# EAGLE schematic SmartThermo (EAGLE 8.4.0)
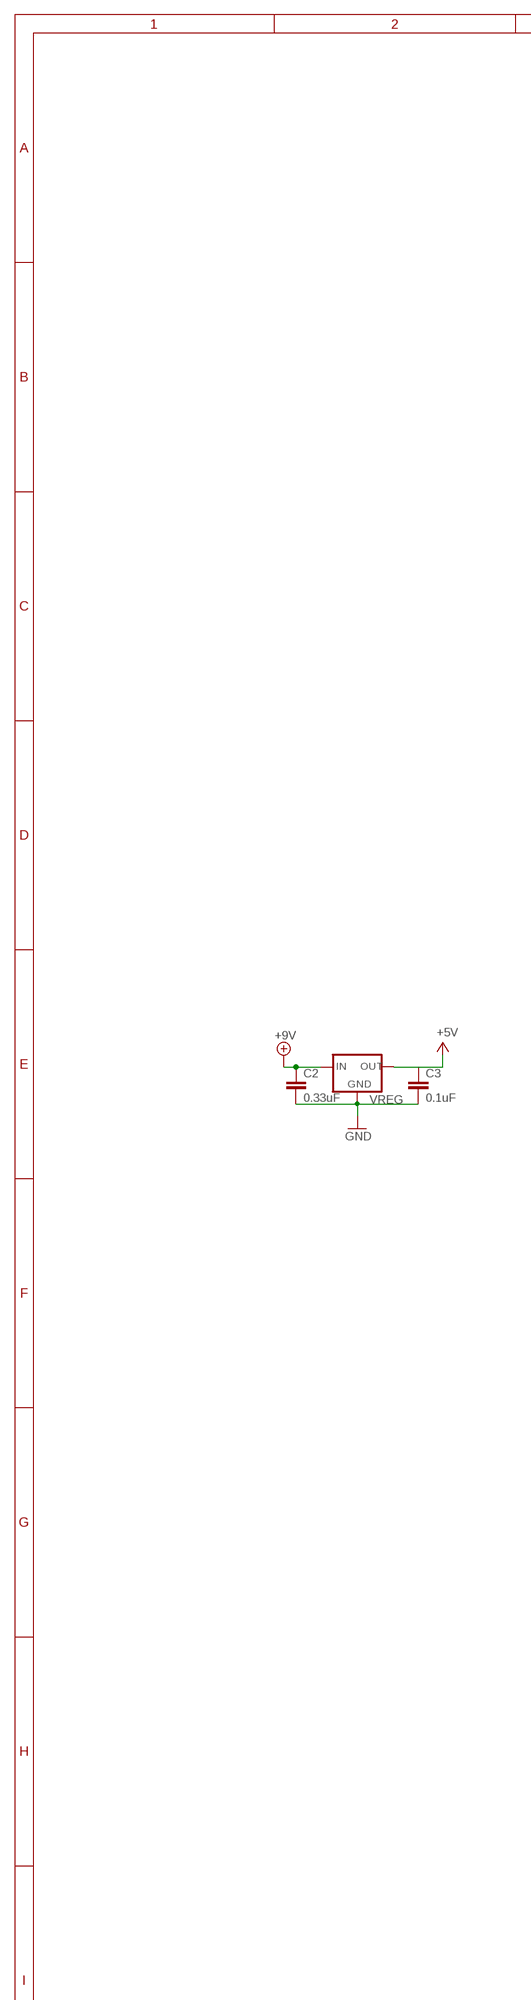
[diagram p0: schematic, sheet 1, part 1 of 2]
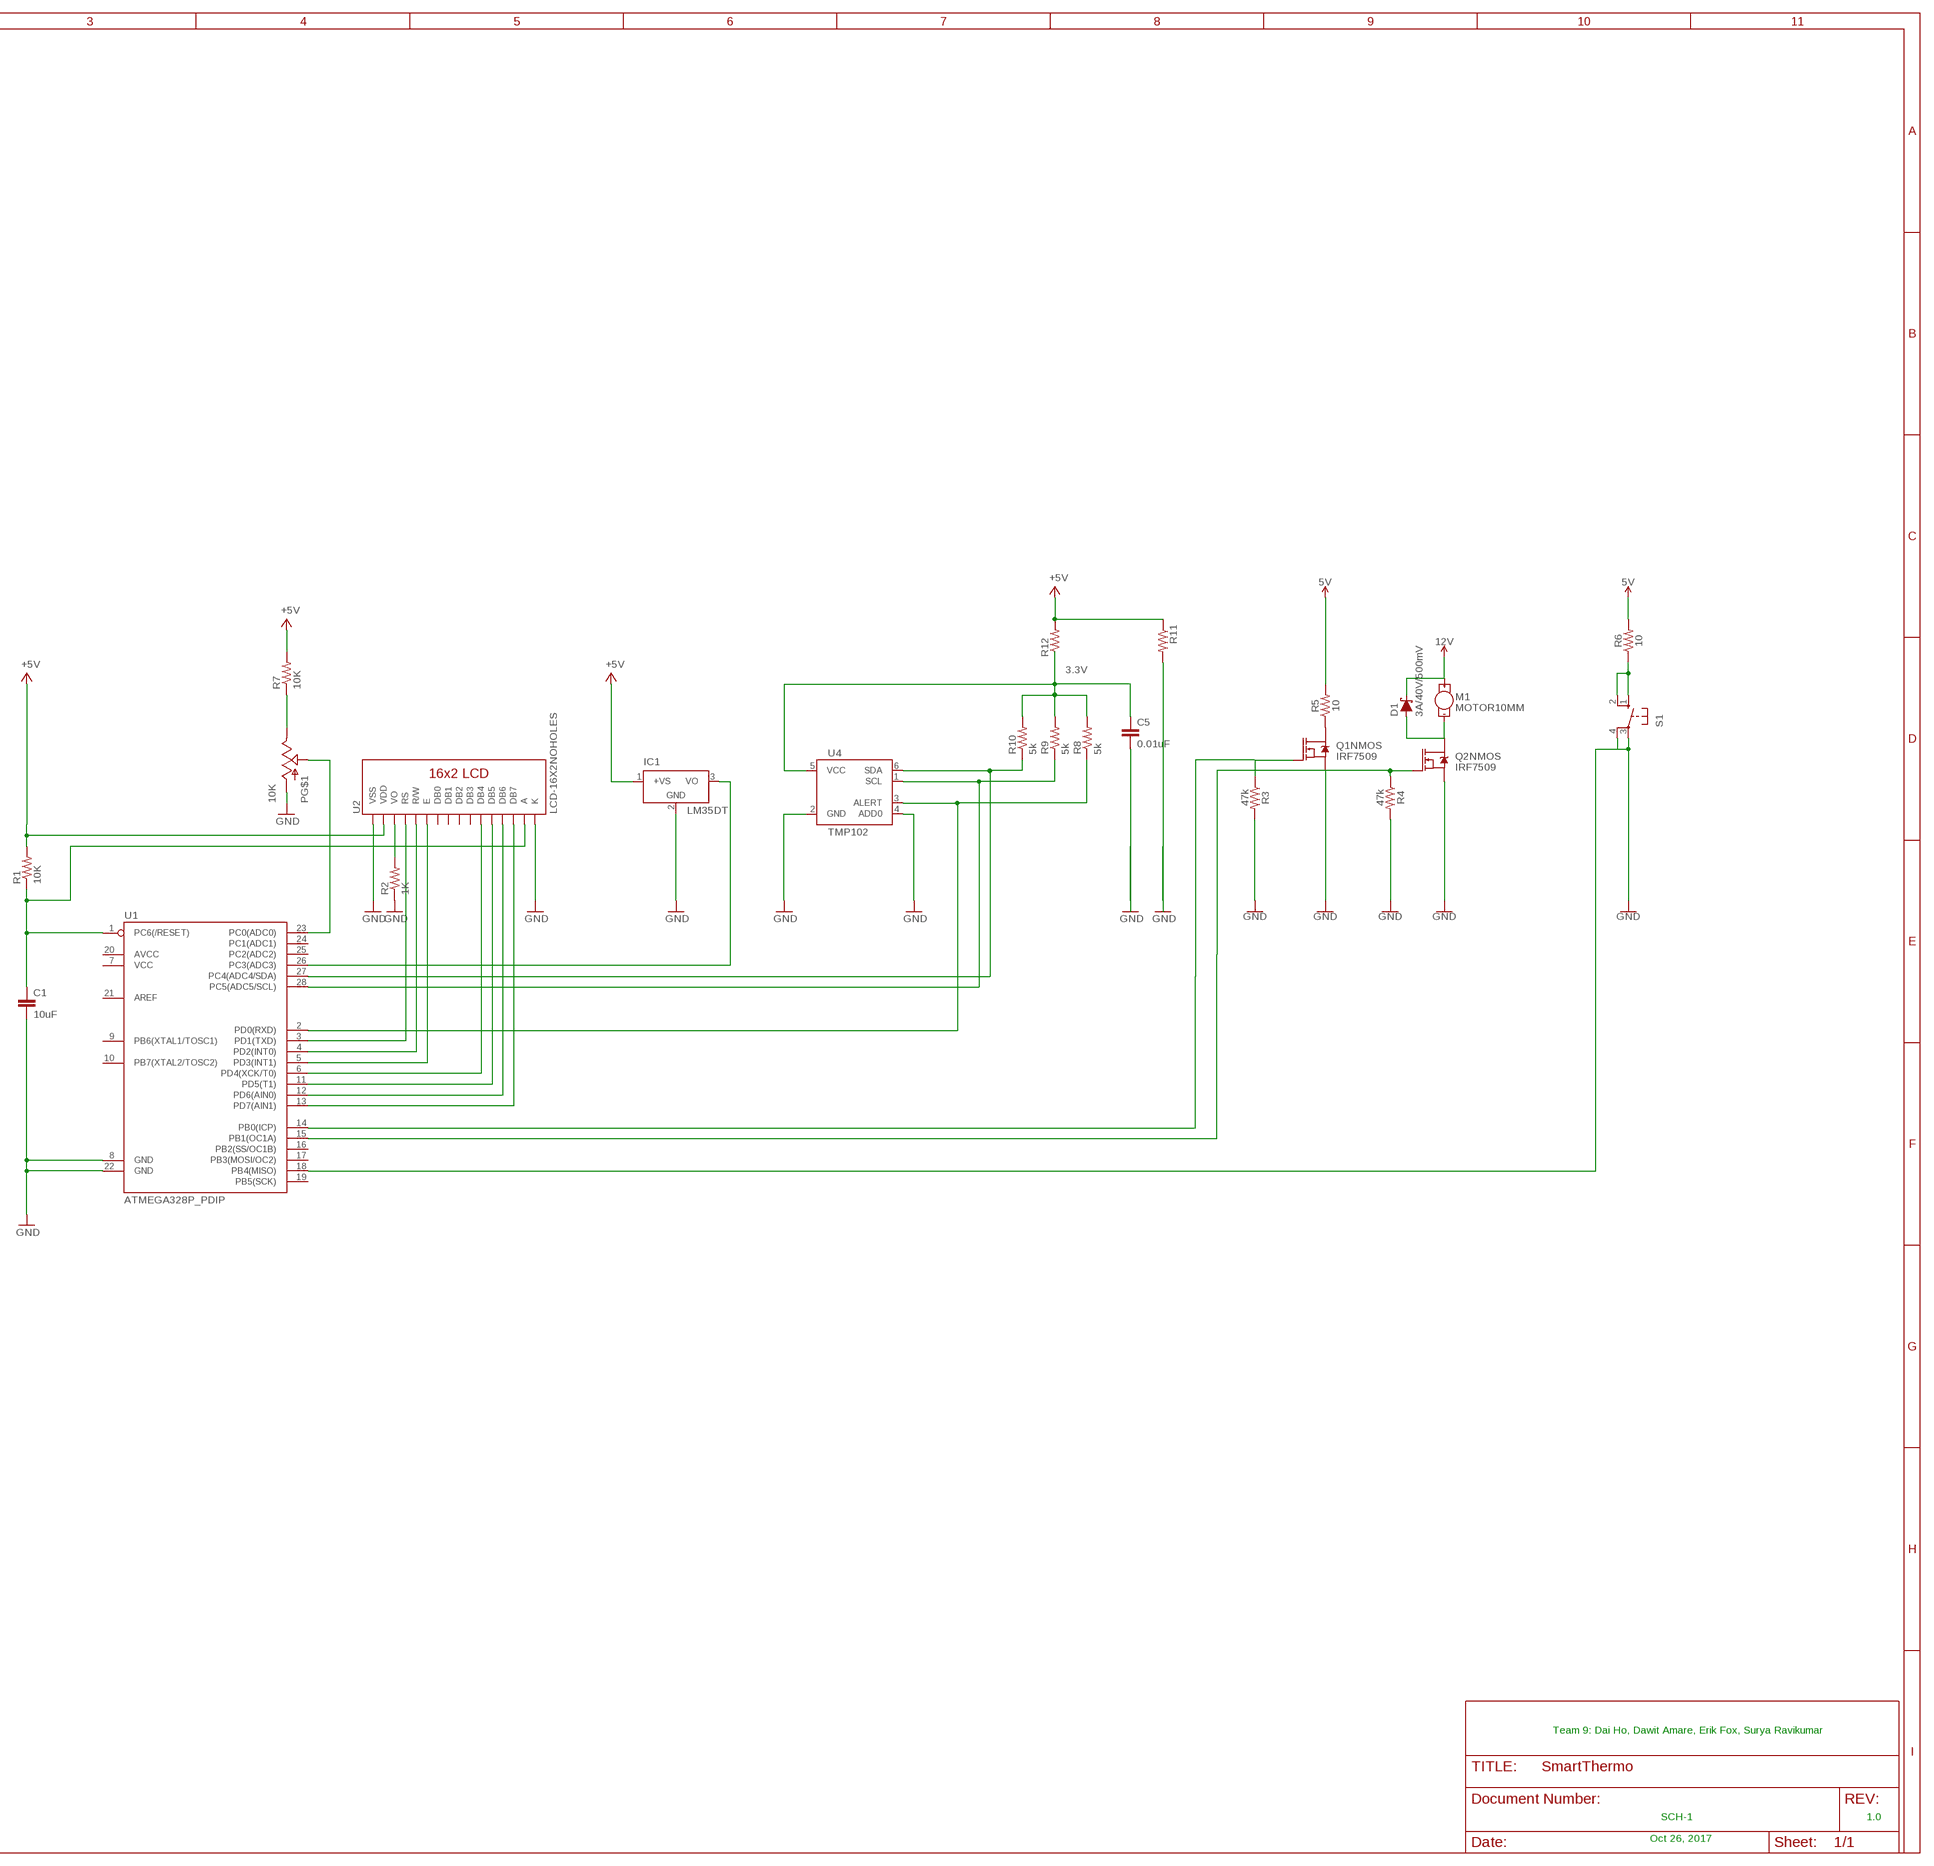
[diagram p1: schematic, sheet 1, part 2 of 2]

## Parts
C1  10uF  10UF-6.3V-20%(1206)  [1206]
C2  0.33uF  C7.5/3  [C7.5B3]
C3  0.1uF  C7.5/3  [C7.5B3]
C5  0.01uF  C2,5-3  [C2.5-3]
D1  3A/40V/500mV  DIODE-SCHOTTKY-B340A  [SMA-DIODE]
IC1  LM35DT  [TO220V]
M1  MOTOR10MM  [VIBE-MOTOR-10MM]
P  10K  POT_SWITCHPOT_PTH  [POT_PTH]
Q1  IRF7509  [MSOP8]
Q2  IRF7509  [MSOP8]
R1  10K  RESISTOR1206  [1206]
R2  1K  1KOHM1/10W1%(0603)  [0603-RES]
R3  47k  47KOHM-0603-1/10W-1%  [0603]
R4  47k  47KOHM-0603-1/10W-1%  [0603]
R5  10  10OHM-0603-1/10W-5%  [0603]
R6  10  10OHM-0603-1/10W-5%  [0603]
R7  10K  RESISTOR1206  [1206]
R8  5k  R-US_0204/5  [0204/5]
R9  5k  R-US_0204/5  [0204/5]
R10  5k  R-US_0204/5  [0204/5]
R11  R-US_0204/5  [0204/5]
R12  R-US_0204/5  [0204/5]
S1  10-XX  [B3F-10XX]
U1  ATMEGA328P_PDIP  [DIL28-3]
U2  LCD-16X2NOHOLES  [LCD-16X2_NOHOLES]
U4  TMP102  [SOT563]
VREG  V_REG_78XX-TO-220  [TO-220-ALT]

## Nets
3.3V: C5.1 R10.2 R12.1
5V: R5.2 R6.2
12V: D1.C M1.+
+9V: C2.1 VREG.IN
GND: C1.2 C2.2 C3.2 IC1.2(GND) P.E@1(A) Q1.1(NMOS:S) Q2.1(NMOS:S) R2.1 R3.2 R4.2 S1.3(P) S1.4(P1) U1.8(GND) U1.18(PB4(MISO)) U1.22(GND) U2.1(VSS) U2.16(K) U4.2(GND) U4.4(ADD0)
N$1: C1.1 R1.1 U1.1(PC6(/RESET)) U2.15(A)
N$2: IC1.3(VO) U1.26(PC3(ADC3))
N$3: Q1.2(NMOS:G) R3.1 U1.14(PB0(ICP))
N$4: Q2.2(NMOS:G) R4.1 U1.15(PB1(OC1A))
N$5: U1.3(PD1(TXD)) U2.4(RS)
N$6: U1.4(PD2(INT0)) U2.5(R/W)
N$7: U1.5(PD3(INT1)) U2.6(E)
N$8: U1.6(PD4(XCK/T0)) U2.11(DB4)
N$9: U1.11(PD5(T1)) U2.12(DB5)
N$10: U1.12(PD6(AIN0)) U2.13(DB6)
N$11: U1.13(PD7(AIN1)) U2.14(DB7)
N$12: R9.2
N$13: D1.A M1.- Q2.7(NMOS:D) Q2.8(NMOS:D)
N$14: Q1.7(NMOS:D) Q1.8(NMOS:D) R5.1
N$15: R6.1 S1.1(S) S1.2(S1)
N$16: R2.2 U2.3(VO)
N$17: P.E@2(E) R7.1
N$18: P.WAND(S) U1.23(PC0(ADC0))
N$22: R8.2
N$23: R10.1 U1.27(PC4(ADC4/SDA)) U4.6(SDA)
N$24: R9.1 U1.28(PC5(ADC5/SCL)) U4.1(SCL)
N$25: R8.1 U1.2(PD0(RXD)) U4.3(ALERT)
N$26: R11.2
N$27: C5.2
V+: IC1.1(+VS) R1.2 R7.2 R11.1 R12.2 U2.2(VDD) VREG.OUT ; supply symbol labelled +5V
Unconnected: C3.1 P.S1 P.S2 Q1.3(PMOS:S) Q1.4(PMOS:G) Q1.5(PMOS:D) Q1.6(PMOS:D) Q2.3(PMOS:S) Q2.4(PMOS:G) Q2.5(PMOS:D) Q2.6(PMOS:D) U1.7(VCC) U1.9(PB6(XTAL1/TOSC1)) U1.10(PB7(XTAL2/TOSC2)) U1.16(PB2(SS/OC1B)) U1.17(PB3(MOSI/OC2)) U1.19(PB5(SCK)) U1.20(AVCC) U1.21(AREF) U1.24(PC1(ADC1)) U1.25(PC2(ADC2)) U2.7(DB0) U2.8(DB1) U2.9(DB2) U2.10(DB3) U4.5(VCC) VREG.GND

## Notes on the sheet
- Team 9: Dai Ho, Dawit Amare, Erik Fox, Surya Ravikumar
- SCH-1 | 1.0
- Oct 26, 2017

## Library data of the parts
C1 = SparkFun-Capacitors:10UF-6.3V-20%(1206): CAP-10057; PROD_ID: CAP-10057
C2 C3 C5 = capacitor-wima:C: CAPACITOR
D1 = SparkFun-DiscreteSemi:DIODE-SCHOTTKY: Schottky diode; PROD_ID: DIO-09886
IC1 = lm35:LM35: Single-Supply Centigrade Temperature Sensor Vout = (10mV/°C x Temp °C) +5mmmV Source: http://www.national.com/ds/LM/LM35.pdf
M1 = SparkFun-Electromechanical:MOTOR: Motor (Single-Phase); PROD_ID: COMP-08572; SF_SKU: ROB-08449
P = button_TestFootprint:POT_SWITCH: Potentiometer w/ switch.
Q1 Q2 = SparkFun-DiscreteSemi:IRF7509: Dual N and P Channel MOSFET Dual N/P-Channel 30V 1.25 W 7.8/7.5 nC Hexfet Power Mosfet Surface Mount-MICRO-8. NMOS RDS(ON) 0.11Ω. PMOS RDS(ON) 0.20Ω. Link to datasheet SparkFun Products: SparkFun RedBot Mainboard SparkFun Wake on Shake; PROD_ID: TRANS-07913
R1 R7 = SparkFun-Passives:RESISTOR: Resistor
R2 = SparkFun-Resistors:1KOHM1/10W1%(0603): RES-07856; PROD_ID: RES-07856
R3 R4 = SparkFun-Resistors:47KOHM: 47kΩ resistor; PROD_ID: RES-07871
R5 R6 = SparkFun-Resistors:10OHM: 10Ω resistor; PROD_ID: RES-09834
R8-R12 = resistor:R-US_: RESISTOR, American symbol
S1 = switch-omron:10-XX: OMRON SWITCH; MPN: B3F-1000; OC_FARNELL: 176432; OC_NEWARK: 36M3542
U1 = SparkFun-DigitalIC:ATMEGA328P_PDIP: uC used in the Arduino 32kb flash, 1k EEPROM, 2k SRAM This is the through-hole version of this chip.
U2 = SparkFun-Displays:LCD-16X2: Standard text-only 16x2 parallel input LCD
U4 = SparkFun-Sensors:TMP102: I2C degC temp sensor
VREG = SparkFun-PowerIC:V_REG_78XX: Voltage Regulator Standard 7805 5V regulator. IGO (Input Ground Output). Spark Fun Electronics SKU : COM-00107

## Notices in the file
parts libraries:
SparkFun-DigitalIC: Licensing: Creative Commons ShareAlike 4.0 International - https://creativecommons.org/licenses/by-sa/4.0
